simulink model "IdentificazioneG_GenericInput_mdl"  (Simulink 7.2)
settings: Solver=ode45  StartTime=0.0  StopTime=100  RelTol=1e-3
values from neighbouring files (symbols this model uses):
  Ts = 0.1    [IdentificazioneG.m]
undefined symbols (not defined in the file or in its folder): A
libraries: simulink x1, cstblocks x1

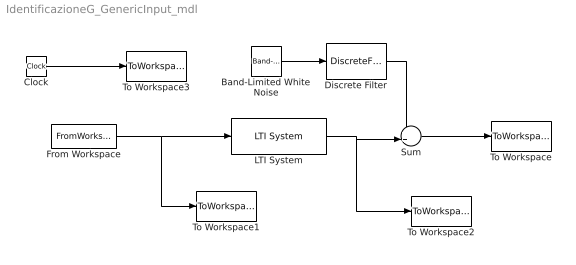
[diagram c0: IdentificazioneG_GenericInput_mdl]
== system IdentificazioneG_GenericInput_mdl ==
  Band-Limited White Noise : simulink/Sources/Band-Limited White Noise  SystemSampleTime=-1  Cov=NP  Ts=Ts  seed=[23341]
  Clock : Clock
  Discrete Filter : DiscreteFilter  Denominator=A  SampleTime=Ts
  From Workspace : FromWorkspace  VariableName=[timed ui]  SampleTime=0
  LTI System : cstblocks/LTI System  SystemSampleTime=-1  sys=G  IC=[]
  Sum : Sum  Inputs=++|  OutDataType=sfix(16)  OutScaling=2^0
  To Workspace : ToWorkspace  VariableName=yn  SampleTime=Ts  SaveFormat=Array
  To Workspace1 : ToWorkspace  VariableName=u  SampleTime=Ts  SaveFormat=Array
  To Workspace2 : ToWorkspace  VariableName=y  SampleTime=Ts  SaveFormat=Array
  To Workspace3 : ToWorkspace  VariableName=time  SampleTime=-1  SaveFormat=Array
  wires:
  From Workspace/1 -> LTI System/1, To Workspace1/1
  Clock/1 -> To Workspace3/1
  Sum/1 -> To Workspace/1
  LTI System/1 -> Sum/2, To Workspace2/1
  Band-Limited White Noise/1 -> Discrete Filter/1
  Discrete Filter/1 -> Sum/1
